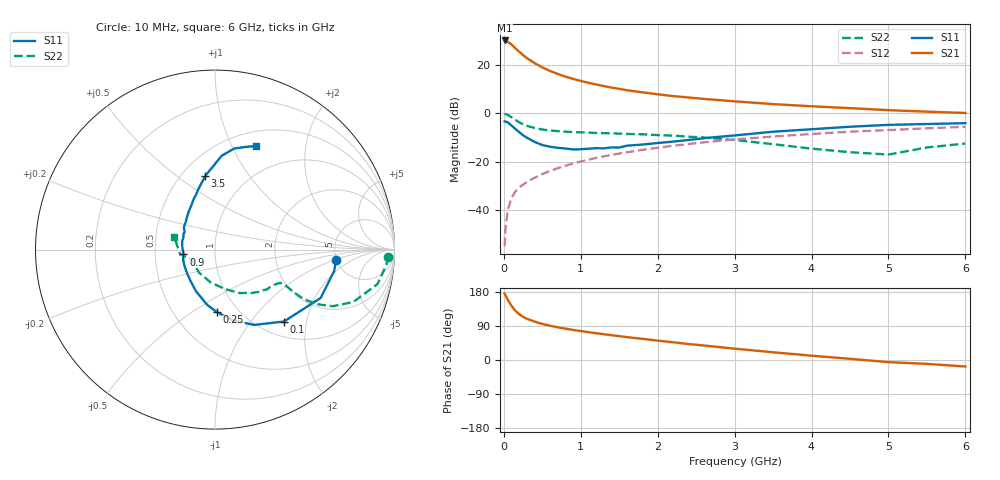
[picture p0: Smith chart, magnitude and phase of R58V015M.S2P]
! SIEMENS Small Signal Semiconductors
! BFR183
! Si NPN RF Bipolar Junction Transistor in SOT23
! VCE = 8 V  IC = 15 mA
! Common Emitter S-Parameters:  May  1996
# GHz  S  MA  R  50
!  f  S11  S21  S12  S22
! GHz  MAG  ANG  MAG  ANG  MAG  ANG  MAG  ANG
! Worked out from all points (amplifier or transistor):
!   36 points, 10 MHz to 6 GHz, reference 50 ohm
!   highest |S21| = 30.0 dB at 10 MHz (marker M1)
!   |S21| within 3 dB of that: start of sweep to 143.2 MHz
!   unconditionally stable (mu >= 1): 707.7 MHz to 2.549 GHz
!   at 250 MHz: K = 0.71, MSG = 26.7 dB, |S12| = -29.5 dB
!   at 1.4 GHz: K = 1.05, MAG = 12.6 dB, |S12| = -17.3 dB
!   at 6 GHz: K = 0.89, MSG = 2.9 dB, |S12| = -5.6 dB
!   S11 on the Smith chart (normalised r, x): 10 MHz: 4.95, -1.08; 100 MHz: 1.28, -1.48; 250 MHz: 0.80, -0.64; 900 MHz: 0.70, -0.04; 3.5 GHz: 0.65, +0.64; 6 GHz: 0.66, +1.24
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0.01  0.6772 -5.0  31.62 175.1  0.0018 86.7  0.9671 -2.3
0.02  0.6745 -10.3  31.05 171.0  0.0039 81.8  0.9592 -5.0
0.05  0.6473 -24.6  29.8 159.5  0.0099 80.5  0.9252 -12.0
0.1  0.5551 -46.2  26.11 142.8  0.0179 71.4  0.8233 -20.8
0.15  0.4727 -62.6  21.85 129.9  0.0242 67.9  0.7254 -25.8
0.2  0.4054 -76.1  18.56 120.9  0.0295 66.1  0.6486 -28.0
0.25  0.3493 -88.0  15.79 113.8  0.0336 66.0  0.5874 -28.9
0.3  0.3113 -98.0  13.69 108.7  0.0378 66.6  0.5466 -29.0
0.4  0.255 -114.5  10.78 101.4  0.0466 67.0  0.4937 -28.3
0.5  0.2198 -129.1  8.782 95.1  0.0552 68.0  0.4595 -27.4
0.6  0.2028 -140.5  7.445 90.4  0.0642 68.4  0.4392 -26.9
0.7  0.193 -151.5  6.462 86.3  0.073 68.7  0.4253 -26.8
0.8  0.1865 -162.2  5.67 82.7  0.082 68.4  0.415 -26.9
0.9  0.1782 -171.3  5.086 79.3  0.0916 68.4  0.4074 -27.1
1.1  0.1846 172.8  4.241 73.5  0.1096 67.7  0.3962 -28.7
1.3  0.1877 159.5  3.613 68.0  0.1285 66.3  0.3864 -30.2
1.6  0.2132 144.4  2.976 60.4  0.1561 63.9  0.3722 -34.0
2.2  0.2584 124.4  2.251 46.8  0.212 58.2  0.343 -43.3
3.5  0.4136 97.6  1.537 20.4  0.329 42.7  0.2288 -75.0
4.5  0.5243 85.9  1.268 3.1  0.4152 30.6  0.1562 -125.1
5.5  0.597 73.4  1.072 -10.2  0.4869 19.1  0.1959 -172.3
6  0.6216 68.4  1.009 -17.2  0.5218 11.7  0.2361 163.3
